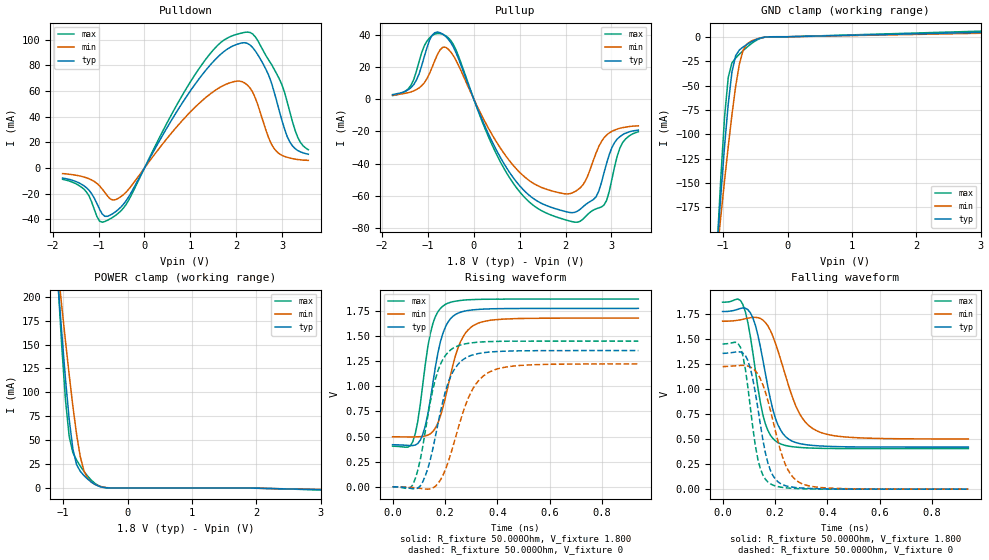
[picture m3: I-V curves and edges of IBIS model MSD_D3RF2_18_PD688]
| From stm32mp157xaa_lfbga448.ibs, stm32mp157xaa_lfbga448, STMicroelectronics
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[Model] MSD_D3RF2_18_PD688
Model_type   I/O
C_comp 2.432pF   2.349pF   2.554pF
Vinh = 1.150V
Vinl = 650.000mV
Vmeas = 900.000mV
Vref = 900.000mV
[Model Spec]
Vinh   1.150V   1.100V   1.200V
Vinl   650.000mV   600.000mV   700.000mV
Vmeas   900.000mV   850.000mV   950.000mV
Vref   900.000mV   850.000mV   950.000mV
[Temperature Range]   25.000   125.000   -40.000
[Voltage Range]   1.800V   1.700V   1.900V
[GND Clamp Reference]   0.00V   0.00V   0.00V
[Pulldown Reference]   0.00V   0.00V   0.00V
[POWER Clamp Reference]   1.800V   1.700V   1.900V
[Pullup Reference]   1.800V   1.700V   1.900V
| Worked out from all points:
|   slope of the pulldown table from 0 to 0.27 V, typ, clamps not added: 15.3 ohm
|   slope of the pullup table from 0 to 0.27 V, typ, clamps not added: 14.6 ohm
|   GND clamp passes 1 mA (typ) near -0.40 V on its own axis
|   POWER clamp passes 1 mA (typ) near -0.41 V on its own axis
|   rising waveform, R_fixture 50.000Ohm, V_fixture 1.800: 20-80 % time 57.7ps typ, 73.1ps min, 50.3ps max; typ from 0.418 V to 1.77 V
|   rising waveform, R_fixture 50.000Ohm, V_fixture 0: 20-80 % time 75.4ps typ, 95ps min, 66.7ps max; typ from 0.001 V to 1.35 V
|   falling waveform, R_fixture 50.000Ohm, V_fixture 1.800: 20-80 % time 66.5ps typ, 94.2ps min, 56ps max; typ from 1.77 V to 0.419 V
|   falling waveform, R_fixture 50.000Ohm, V_fixture 0: 20-80 % time 55.6ps typ, 77.8ps min, 46.5ps max; typ from 1.35 V to 0 V
[GND Clamp]
-1.785V   -902.9mA   -690.2mA   -1.212A
-1.094V   -215.4mA   -221.6mA   -216.3mA
-1.036V   -162.5mA   -184.2mA   -144.3mA
-978.8mV  -112.8mA   -147.8mA   -82.88mA
-921.2mV  -69.08mA   -112.8mA   -41.72mA
-863.6mV  -36.25mA   -80.05mA   -26.83mA
-806.1mV  -19.45mA   -51mA      -21.84mA
-748.5mV  -13.61mA   -28.13mA   -17.96mA
-690.9mV  -10.53mA   -14.07mA   -14.3mA
-575.8mV  -5.725mA   -4.911mA   -7.736mA
-287.9mV  -77.18uA   -128.3uA   -62.8uA
3.57V     5.336mA    4.258mA    6.829mA
[Power Clamp]
-1.77V    884.4mA    691.3mA    1.161A
-1.079V   213.2mA    227.2mA    213.2mA
-1.021V   161.7mA    189.9mA    147.7mA
-963.6mV  113.6mA    153.5mA    91.76mA
-906.1mV  71.75mA    118.3mA    53.67mA
-848.5mV  40.54mA    85.21mA    36.83mA
-790.9mV  24.24mA    55.8mA     29.06mA
-733.3mV  17.36mA    32.54mA    22.8mA
-618.2mV  9.196mA    9.941mA    12.25mA
-503mV    3.543mA    3.631mA    4.61mA
-272.7mV  33uA       105.9uA    31.94uA
3.585V    -2.704mA   -2.298mA   -3.251mA
[Pulldown]
-1.785V   -7.9mA     -4.4mA     -8.8mA
-1.267V   -15.3mA    -7.6mA     -18.6mA
-978.8mV  -32.1mA    -13.9mA    -41.43mA
-575.8mV  -32.49mA   -23.76mA   -35.4mA
1.209V    70.38mA    50.93mA    78.44mA
1.67V     88.85mA    63.31mA    97.99mA
2.188V    97.58mA    66.1mA     105.7mA
2.476V    87.79mA    48.5mA     98.79mA
2.821V    59.7mA     15.3mA     77.19mA
3.167V    20.3mA     7.8mA      43.7mA
3.339V    13.6mA     6.6mA      23.9mA
3.57V     10.7mA     5.9mA      14.2mA
[Pullup]
-1.77V    2.8mA      2.5mA      2.179mA
-1.367V   7.2mA      4.468mA    8.689mA
-1.136V   20.6mA     8.305mA    28.74mA
-906.1mV  39.6mA     19.85mA    39.38mA
-618.2mV  38.98mA    32.14mA    39.33mA
878.8mV   -49.37mA   -41.66mA   -52.88mA
1.455V    -64.24mA   -54.44mA   -68.75mA
2.203V    -70.07mA   -57.29mA   -76.21mA
2.664V    -60.51mA   -33.36mA   -67.93mA
2.836V    -45.7mA    -23.98mA   -65.63mA
3.182V    -23.3mA    -18.03mA   -30.43mA
3.585V    -19.2mA    -16.53mA   -20.22mA
[Ramp]
R_load=50.000Ohm
dV/dt_r   811.440mV/67.000ps  718.679mV/85.000ps  872.070mV/58.500ps
dV/dt_f   811.440mV/62.000ps  718.679mV/86.500ps  872.070mV/52.000ps
[Rising waveform]
R_fixture=50.000Ohm
V_fixture=1.800
V_fixture_min=1.700
V_fixture_max=1.900
0s        418.5mV    497.4mV    403.8mV
68ps      410.3mV    495.6mV    408.3mV
87ps      415.6mV    496.2mV    532.1mV
106ps     464.7mV    498.8mV    823.5mV
144ps     865.1mV    526.3mV    1.521V
173ps     1.328V     634mV      1.738V
202ps     1.589V     889.8mV    1.812V
259ps     1.733V     1.439V     1.85V
326ps     1.761V     1.624V     1.861V
938ps     1.772V     1.675V     1.864V
[Rising waveform]
R_fixture=50.000Ohm
V_fixture=0
0s        1.108mV    972.7uV    969.2uV
77ps      -18.47mV   -6.677mV   20.17mV
115ps     48.9mV     -18.24mV   397.2mV
144ps     269mV      -20.17mV   841.9mV
173ps     623.7mV    32.51mV    1.152V
202ps     949.6mV    174.2mV    1.305V
230ps     1.141V     397mV      1.375V
298ps     1.303V     932.9mV    1.428V
374ps     1.339V     1.145V     1.442V
938ps     1.353V     1.22V      1.447V
[Falling waveform]
R_fixture=50.000Ohm
V_fixture=1.800
V_fixture_min=1.700
V_fixture_max=1.900
0s        1.77V      1.673V     1.863V
68ps      1.8V       1.687V     1.881V
87ps      1.803V     1.698V     1.767V
115ps     1.711V     1.711V     1.369V
144ps     1.422V     1.701V     866.5mV
163ps     1.159V     1.662V     653.8mV
211ps     642mV      1.381V     465mV
288ps     457.9mV    781.8mV    417.1mV
365ps     431.8mV    574.9mV    407.5mV
938ps     419.3mV    500mV      404mV
[Falling waveform]
R_fixture=50.000Ohm
V_fixture=0
0s        1.352V     1.221V     1.446V
68ps      1.367V     1.233V     1.415V
96ps      1.286V     1.227V     1.028V
115ps     1.103V     1.204V     622.7mV
135ps     801.4mV    1.145V     294.3mV
163ps     367.3mV    969.9mV    100.8mV
183ps     184.8mV    781.4mV    52.34mV
240ps     34.65mV    243.8mV    14.1mV
307ps     10.65mV    49.83mV    3.952mV
938ps     2.816uV    29.67uV    3.049uV
